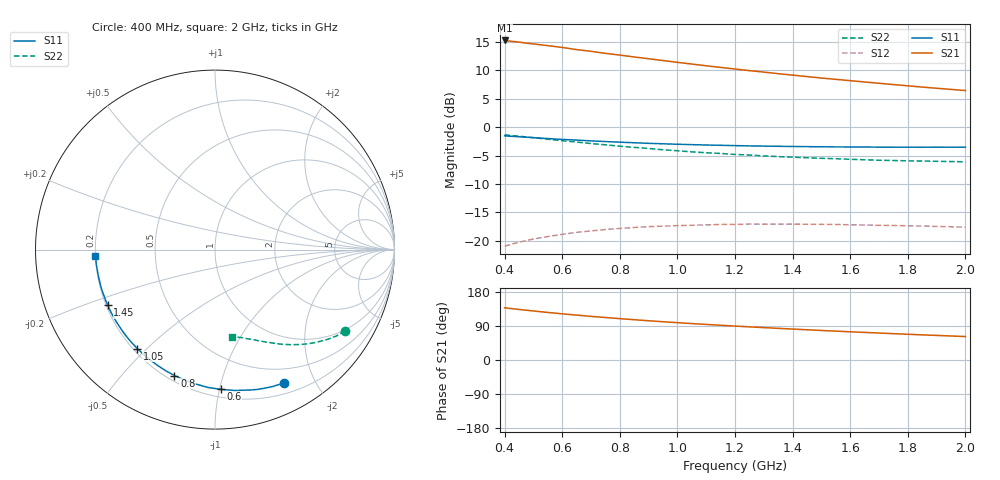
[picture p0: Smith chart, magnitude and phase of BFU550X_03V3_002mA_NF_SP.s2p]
! Filename:  P:\Prog\Test\Noise\ATS_data\Testdata_Net\BFU550X no attenuator noise\BFU550X_APG2013_44_C05_03p3V_002mA_NF_CM01_D.sf
! Date/Time: Fri 26/Jul/2013 14:37:10
! BFU550X_APG2013_44_C05_03p3V_1to10mA_NF_CM01_Bias2_R.sf
! Noise Parameter Data File
! BFU550X_APG2013_44_C05_03p3V_1to10mA_NF_CM01
! Date/time: Wed Jul 24 15:50:55 2013
! VAR V_out= 3.300000
! VAR I_out= 1.995000
! VAR V_in= 0.794900
! VAR I_in= 0.022005
! Device data file deembeded for feedlines and parallel
! Original file: \BFU550X no attenuator noise\BFU550X_APG2013_44_C05_03p3V_002mA_NF_CM01_R.sf
! Feed-files: PR005V01_100713_Feed1.s2p, PR005V01_100713_Feed2.s2p
! Parallel-file: PR005V01_100713_Par.s2p
# MHz S MA R 50
!  Freq-MHz  S11-mag  S11-arg  S21-mag  S21-arg  S12-mag  S12-arg  S22-mag  S22-arg
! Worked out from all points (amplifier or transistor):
!   37 points, 400 MHz to 2 GHz, reference 50 ohm
!   highest |S21| = 15.2 dB at 400 MHz (marker M1)
!   |S21| within 3 dB of that: start of sweep to 865.8 MHz
!   unconditionally stable (mu >= 1): nowhere
!   at 500 MHz: K = 0.16, MSG = 17.1 dB, |S12| = -19.7 dB
!   at 1.1 GHz: K = 0.34, MSG = 14.0 dB, |S12| = -17.2 dB
!   at 2 GHz: K = 0.63, MSG = 12.0 dB, |S12| = -17.6 dB
!   lowest NFmin = 0.53 dB at 460 MHz
!   S11 on the Smith chart (normalised r, x): 400 MHz: 0.32, -1.60; 600 MHz: 0.25, -1.01; 800 MHz: 0.23, -0.70; 1.05 GHz: 0.22, -0.47; 1.45 GHz: 0.21, -0.23; 2 GHz: 0.20, -0.02
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400  0.8369 -62.7  5.768 137.7  0.08994 54.1  0.857 -32.1
420  0.8304 -65.3  5.685 135.9  0.09288 52.8  0.844 -33.4
440  0.8252 -68.1  5.621 134.3  0.09601 51.4  0.8369 -34.4
500  0.807 -75.7  5.375 129.4  0.1039 47.4  0.8078 -38.0
550  0.7928 -81.9  5.194 125.5  0.1093 44.3  0.7817 -40.7
600  0.7792 -87.7  5.008 121.9  0.1143 41.5  0.7591 -43.1
650  0.769 -92.9  4.797 118.5  0.119 39.0  0.7387 -45.2
700  0.7564 -98.3  4.631 115.1  0.1224 36.4  0.7168 -47.5
750  0.7464 -103.0  4.442 112.1  0.126 34.3  0.6987 -49.2
800  0.737 -107.8  4.29 109.1  0.1287 32.1  0.6796 -51.2
850  0.7285 -112.3  4.13 106.3  0.1313 30.1  0.6635 -52.8
900  0.7198 -116.6  3.985 103.5  0.1335 28.2  0.649 -54.4
950  0.7132 -120.6  3.842 101.0  0.1347 26.4  0.6319 -56.2
1050  0.7013 -128.1  3.579 96.2  0.1372 23.3  0.6057 -59.0
1100  0.6959 -131.6  3.455 93.9  0.1384 21.9  0.5948 -60.2
1200  0.6875 -138.2  3.237 89.5  0.1397 19.1  0.5753 -62.7
1300  0.6807 -144.3  3.041 85.5  0.1402 16.8  0.5584 -65.1
1450  0.6734 -152.5  2.778 79.8  0.1401 13.6  0.5376 -68.2
1500  0.6716 -155.2  2.698 78.0  0.1399 12.7  0.532 -69.3
1600  0.6693 -160.1  2.557 74.5  0.1386 11.0  0.5212 -71.4
1750  0.6663 -166.9  2.364 69.5  0.1366 8.9  0.5087 -74.2
2000  0.6667 -177.1  2.095 61.9  0.132 6.3  0.4956 -78.8
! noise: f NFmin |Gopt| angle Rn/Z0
400  0.5845  0.4735  30.08  0.1919
460  0.531  0.4674  40.82  0.1625
600  0.6293  0.4808  48.39  0.19
800  0.6789  0.4757  68.52  0.1529
1000  0.7512  0.4804  83.98  0.1374
1200  0.7769  0.5068  97.84  0.1253
1400  0.834  0.51  111.7  0.1158
1600  0.8226  0.4932  126.5  0.0841
1800  0.8328  0.5432  141.7  0.0582
2000  0.9309  0.602  150.9  0.0469
